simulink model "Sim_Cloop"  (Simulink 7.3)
settings: Solver=ode45  StartTime=0.0  StopTime=40  RelTol=1e-3
InitFcn:
  | run
StopFcn:
  | Pl
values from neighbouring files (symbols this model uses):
  Acl = [    [closedloop.m]    (also in closedloop_eo.m)
  Bcl = [    [closedloop.m]    (also in closedloop_eo.m)
  Ccl = [    [closedloop.m]    (also in closedloop_eo.m)
  d2r = pi/180    (= 0.0174532925199)    [run.m]
  Dcl = [    [closedloop.m]    (also in closedloop_eo.m)
  LBThrust = 0.96097e+6    (= 960970)    [run.m]

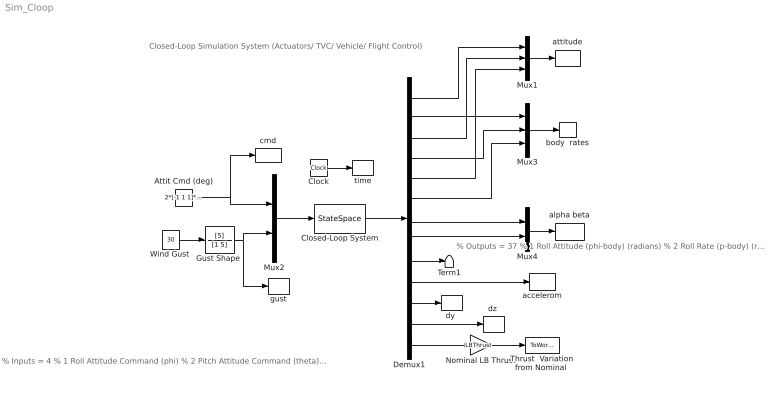
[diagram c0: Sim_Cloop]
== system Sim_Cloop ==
  note: Closed-Loop Simulation System (Actuators/ TVC/ Vehicle/ Flight Control)
  note: % Inputs = 4 % 1 Roll Attitude Command (phi) % 2 Pitch Attitude Command (theta) % 3 Yaw Attitude Command (psi) % 4 Wind Gust Velocity (ft/sec)
  note: % Outputs = 37 % 1 Roll Attitude (phi-body) (radians) % 2 Roll Rate (p-body) (rad/sec) % 3 Pitch Attitude (thet-bdy) (radians) % 4 Pitch Rate (q-body) (rad/sec) % 5 Yaw Attitude (psi-body) (radians) % 6 Yaw Rate (r-body) (rad/sec) % 7 Angle of attack, alfa, (radians) % 8 Angle of sideslip, beta, (radian) % 9 Change in Altitude, delta-h, (feet) % 10 Forward Acceleration (V-dot) (ft/sec) % 11 Cross Range Velocity (Vcr) (ft/sec) % 12 Accelerom # 1, (along Z), (ft/sec^2) Translat. Acceler % 13 Accelerom # 2, (along Y), (ft/sec^2) Translat. Acceler % 14 Engine-1 Pitch Deftect (rad) % 15 Engine-2 Pitch Deftect (rad) % 16 Engine-3 Pitch Deftect (rad) % 17 Engine-4 Pitch Deftect (rad) % 18 Engine-5 Pitch Deftect (rad) % 19 Engine-6 Pitch Deftect (rad) % 20 Engine-7 Pitch Deftect (rad) % 21 Engine-8 Pitch Deftect (rad) % 22 Engine-9 Pitch Deftect (rad) % 23 Engine-1 Yaw Deftect (rad) % 24 Engine-2 Yaw Deftect (rad) % 25 Engine-3 Yaw Deftect (rad) % 26 Engine-4 Yaw Deftect (rad) % 27 Engine-5 Yaw Deftect (rad) % 28 Engine-6 Yaw Deftect (rad) % 29 Engine-7 Yaw Deftect (rad) % 30 Engine-8 Yaw Deftect (rad) % 31 Engine-9 Yaw Deftect (rad) % 32 Engine-4 Throttle % 33 Engine-5 Throttle % 34 Engine-6 Throttle % 35 Engine-7 Throttle % 36 Engine-8 Throttle % 37 Engine-9 Throttle
  Attit Cmd (deg) : Constant  Value=2*[-1 1 1]*d2r  OutDataType=sfix(16)  OutScaling=2^0
  Clock : Clock
  Closed-Loop System : StateSpace  A=Acl  B=Bcl  C=Ccl  D=Dcl
  Demux1 : Demux  Outputs="[1,1,1,1,1,1,1,1,  3, 2, 9, 9, 6]"
  "Gust Shape " : TransferFcn  Numerator=[5]  Denominator=[1 5]
  Mux1 : Mux  Inputs=3
  Mux2 : Mux  Inputs=[3, 1]
  Mux3 : Mux  Inputs=3
  Mux4 : Mux  Inputs=2
  Nominal LB Thrust : Gain  Gain=LBThrust  ParameterDataType=sfix(16)  ParameterScaling=2^0  OutDataType=sfix(16)  OutScaling=2^0
  Term1 : Terminator
  "Thrust  Variation from Nominal " : ToWorkspace  VariableName=Dthrust  SampleTime=-1  SaveFormat=Array
  "Wind Gust " : Constant  Value=30  OutDataType=sfix(16)  OutScaling=2^0
  accelerom : ToWorkspace  VariableName=accel  SampleTime=-1  SaveFormat=Array
  alpha beta : ToWorkspace  VariableName=albet  SampleTime=-1  SaveFormat=Array
  attitude : ToWorkspace  VariableName=attit  SampleTime=-1  SaveFormat=Array
  body  rates : ToWorkspace  VariableName=wb  SampleTime=-1  SaveFormat=Array
  cmd : ToWorkspace  VariableName=cmd  SampleTime=-1  SaveFormat=Array
  "dy " : ToWorkspace  VariableName=dy  SampleTime=-1  SaveFormat=Array
  "dz " : ToWorkspace  VariableName=dz  SampleTime=-1  SaveFormat=Array
  gust : ToWorkspace  VariableName=Gust  SampleTime=-1  SaveFormat=Array
  time : ToWorkspace  VariableName=time  SampleTime=-1  SaveFormat=Array
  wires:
  Mux2/1 -> Closed-Loop System/1
  Closed-Loop System/1 -> Demux1/1
  Attit Cmd (deg)/1 -> cmd/1, Mux2/1
  "Wind Gust "/1 -> "Gust Shape "/1
  "Gust Shape "/1 -> gust/1, Mux2/2
  Mux1/1 -> attitude/1
  Mux3/1 -> body  rates/1
  Mux4/1 -> alpha beta/1
  Demux1/1 -> Mux1/1
  Demux1/3 -> Mux1/2
  Demux1/5 -> Mux1/3
  Demux1/2 -> Mux3/1
  Demux1/4 -> Mux3/2
  Demux1/6 -> Mux3/3
  Demux1/7 -> Mux4/1
  Demux1/8 -> Mux4/2
  Demux1/9 -> Term1/1
  Demux1/10 -> accelerom/1
  Clock/1 -> time/1
  Demux1/11 -> "dy "/1
  Demux1/12 -> "dz "/1
  Nominal LB Thrust/1 -> "Thrust  Variation from Nominal "/1
  Demux1/13 -> Nominal LB Thrust/1
